(* Logix 5000 AddOnInstructionDefinition export A7NETH2P_Generic_Default_IO; software revision 19.01 *)

ADD_ON_INSTRUCTION A7NETH2P_Generic_Default_IO   (* revision 1.0 *)
// Simple interface for generic default IO mapping that uses Input Assembly Instance 150 and Output Assembly Instance 100.
VAR_IN_OUT
   I_Data : INT[2]; {required}   // Input data
   O_Data : INT[2]; {required}   // Output data
        [0]   // Output
END_VAR
VAR_INPUT
   RunStop : BOOL; {access Read Only, required}   // Run (0) or Stop (1)
   Forward : BOOL; {access Read Only, required}   // Run forward direction
   Reverse : BOOL; {required}   // Run reverse direction
   Reset : BOOL; {required}   // Reset the fault
   FrequencyCommand : INT; {access Read Only, required}   // Frequency command/reference
END_VAR
VAR_OUTPUT
   RunningStopped : BOOL; {access Read Only, visible}   // Running (1) or Stopped (0)
   RunningForward : BOOL; {visible}   // Running forward direction
   RunningReverse : BOOL; {visible}   // Running reverse direction
   UpToFrequency : BOOL; {access Read Only, visible}   // Up to frequency
   Alarm : BOOL; {access Read Only, visible}   // Alarm or Trip
   OutputFrequency : INT; {access Read Only, visible}   // Output/feedback frequency
END_VAR

ROUTINE Logic   (* ladder *)
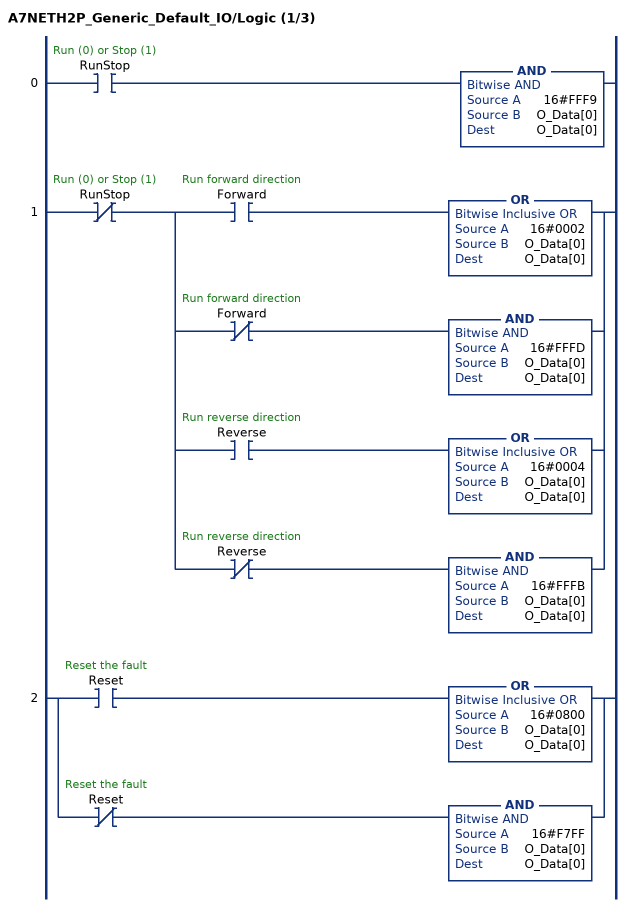
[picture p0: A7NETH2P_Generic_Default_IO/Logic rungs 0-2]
   0: XIC(RunStop)AND(16#FFF9,O_Data[0],O_Data[0]);
   1: XIO(RunStop)[XIC(Forward) OR(16#0002,O_Data[0],O_Data[0]) ,XIO(Forward) AND(16#FFFD,O_Data[0],O_Data[0]) ,XIC(Reverse) OR(16#0004,O_Data[0],O_Data[0]) ,XIO(Reverse) AND(16#FFFB,O_Data[0],O_Data[0]) ];
   2: [XIC(Reset) OR(16#0800,O_Data[0],O_Data[0]) ,XIO(Reset) AND(16#F7FF,O_Data[0],O_Data[0]) ];
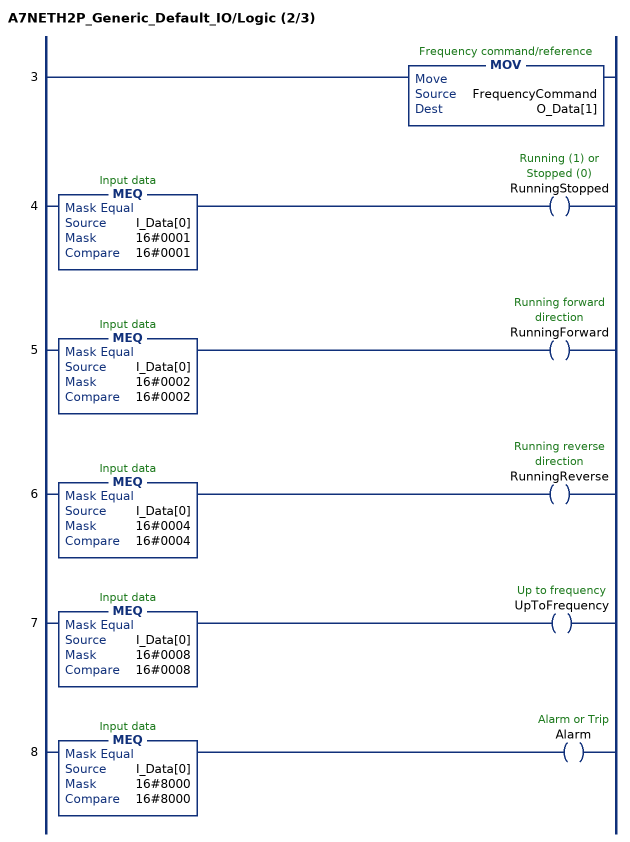
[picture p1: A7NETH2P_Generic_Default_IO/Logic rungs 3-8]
   3: MOV(FrequencyCommand,O_Data[1]);
   4: MEQ(I_Data[0],16#0001,16#0001)OTE(RunningStopped);
   5: MEQ(I_Data[0],16#0002,16#0002)OTE(RunningForward);
   6: MEQ(I_Data[0],16#0004,16#0004)OTE(RunningReverse);
   7: MEQ(I_Data[0],16#0008,16#0008)OTE(UpToFrequency);
   8: MEQ(I_Data[0],16#8000,16#8000)OTE(Alarm);
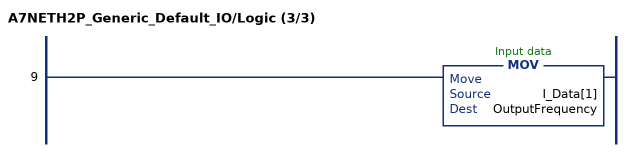
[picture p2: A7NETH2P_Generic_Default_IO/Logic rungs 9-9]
   9: MOV(I_Data[1],OutputFrequency);
END_ROUTINE
END_ADD_ON_INSTRUCTION
